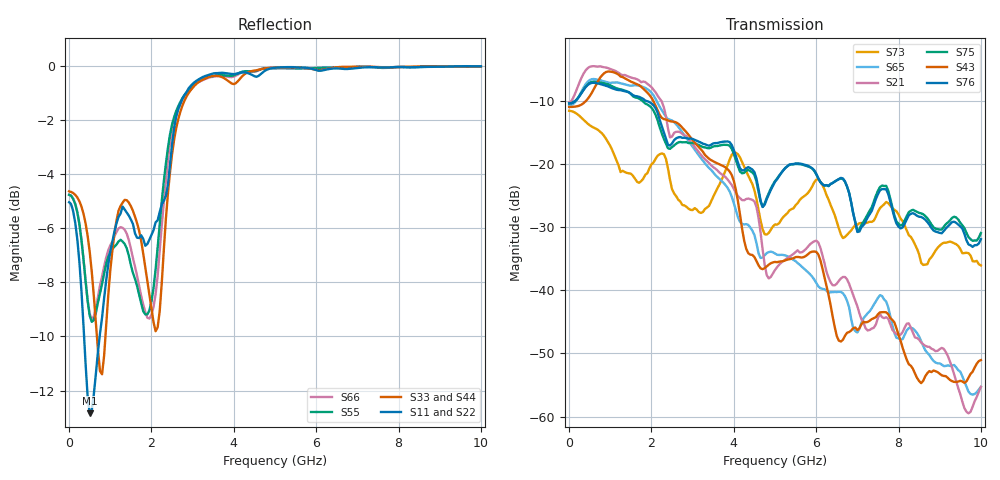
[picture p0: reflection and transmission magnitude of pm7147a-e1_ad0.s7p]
# GHz S DB R 50
! S-Parameters data
! Freq  dbS11  angS11  dbS12  angS12  dbS13  angS13  dbS14  angS14
!  dbS15  angS15  dbS16  angS16  dbS17  angS17  dbS21  angS21
!  dbS22  angS22  dbS23  angS23  dbS24  angS24  dbS25  angS25
!  dbS26  angS26  dbS27  angS27  dbS31  angS31  dbS32  angS32
!  dbS33  angS33  dbS34  angS34  dbS35  angS35  dbS36  angS36
!  dbS37  angS37  dbS41  angS41  dbS42  angS42  dbS43  angS43
!  dbS44  angS44  dbS45  angS45  dbS46  angS46  dbS47  angS47
!  dbS51  angS51  dbS52  angS52  dbS53  angS53  dbS54  angS54
!  dbS55  angS55  dbS56  angS56  dbS57  angS57  dbS61  angS61
!  dbS62  angS62  dbS63  angS63  dbS64  angS64  dbS65  angS65
!  dbS66  angS66  dbS67  angS67  dbS71  angS71  dbS72  angS72
!  dbS73  angS73  dbS74  angS74  dbS75  angS75  dbS76  angS76
!  dbS77  angS77
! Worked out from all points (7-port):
!   279 points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, 1 Hz to 10 GHz, reference 50 ohm
!   strongest paths, dB at 1 Hz, 7.943 MHz, 3.05 GHz, 6.55 GHz, 10 GHz:
!     S76: -10.4, -10.4, -16.1, -22.4, -31.9
!     S43: -10.9, -10.9, -16.6, -48.0, -51.0
!     S75: -10.4, -10.4, -16.7, -22.4, -30.9
!     S21: -10.2, -10.2, -17.3, -38.5, -55.3
!     S65: -10.7, -10.7, -17.7, -40.2, -55.3
!     S73: -11.5, -11.6, -27.0, -30.2, -36.0
!   lowest |S11| = -12.8 dB at 500 MHz (marker M1), VSWR 1.59, Z = 31.5 + j1.35 ohm
!   |S11| at or under -10 dB: 363.5 MHz to 742 MHz (378.4 MHz wide, 68.5 % of centre)
